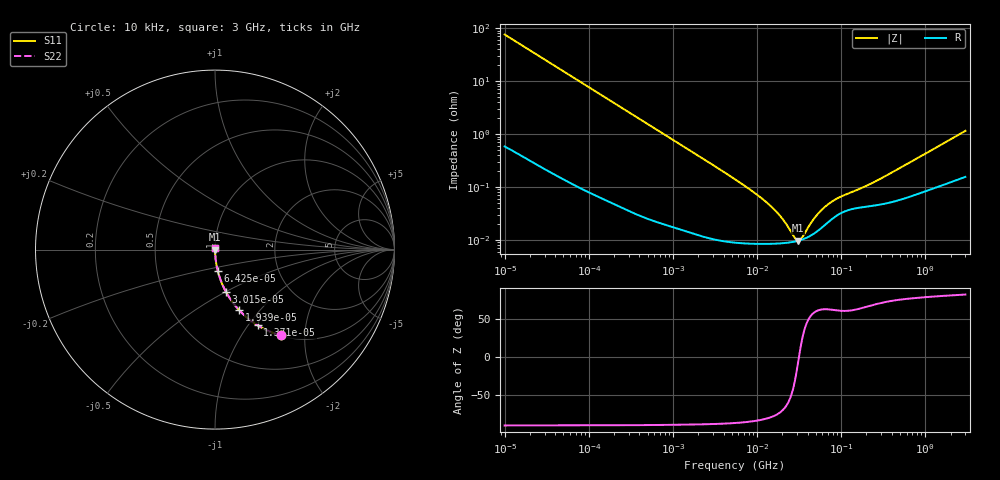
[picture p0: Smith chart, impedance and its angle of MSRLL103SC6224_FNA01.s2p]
! MSRLL103SC6224_FNA01  S-PARAMETER MODEL  ( Standard Model )
! Model Generated by TAIYO YUDEN Corporation (http://www.ty-top.com)
! Version 2.0
! TAIYO YUDEN Control No. 240510
! Copyright(c) 2010 TAIYO YUDEN CO.,LTD. All Rights Reserved.
! Product Description (link to TY-COMPAS)
! https://ds.yuden.co.jp/TYCOMPAS/or/detail?pn=MSRLL103SC6224MFNA01&u=M
! Products Name : Multilayer Ceramic Capacitors
! Characteristics :
!  Capacitance : 0.22 [uF] , Rated Voltage : 10 [V] , TCC : X6S
!  Case Size : 0.52 x 1.0 / 0.02 x 0.039 [mm/inch] , Thickness : 0.3 / 0.012 [mm/inch]
!  (Conditions: Temperature = 25 [degC] , DC Bias Voltage = 0 [V])
! External Node Assignments :
!  1  o---| |---o  2
! GND o---------o GND
! Frequency Range : 10kHz  -  3GHz  [ 401 STEP ]
# MHZ S RI R 50
! Freq[MHz].  S11 Real  S11 Imag  S21 Real  S21 Imag  S12 Real  S12 Imag  S22 Real  S22 Imag
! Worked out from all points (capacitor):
!   401 points, 10 kHz to 3 GHz, reference 50 ohm
!   read as one part in series: C = 210 nF near 10.65 kHz
!   lowest |Z| = 9.75 mohm at 31.02 MHz (marker M1)
!   series resonance near 31.52 MHz, so ESL is about 120 pH
!   S11 on the Smith chart (normalised r, x): 10 kHz: 1.01, -1.52; 13.71 kHz: 1.01, -1.11; 19.39 kHz: 1.01, -0.79; 30.15 kHz: 1.00, -0.51; 64.25 kHz: 1.00, -0.24; 3 GHz: 1.00, +0.02
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0.01  0.3661 -0.4779  0.6339 0.4779  0.6339 0.4779  0.3661 -0.4779
0.013707  0.2368 -0.4211  0.7632 0.4211  0.7632 0.4211  0.2368 -0.4211
0.019389  0.1356 -0.3382  0.8644 0.3382  0.8644 0.3382  0.1356 -0.3382
0.030147  0.062 -0.2368  0.938 0.2368  0.938 0.2368  0.062 -0.2368
0.06425  0.0151 -0.1173  0.9849 0.1173  0.9849 0.1173  0.0151 -0.1173
0.082683  0.00943 -0.0918  0.9906 0.0918  0.9906 0.0918  0.00943 -0.0918
0.199902  0.00196 -0.0385  0.998 0.0385  0.998 0.0385  0.00196 -0.0385
0.683653  0.000341 -0.0114  0.9997 0.0114  0.9997 0.0114  0.000341 -0.0114
5.477226  9.11e-05 -0.0014  0.9999 0.0014  0.9999 0.0014  9.11e-05 -0.0014
9.97066  8.52e-05 -0.000715  0.9999 0.000715  0.9999 0.000715  8.52e-05 -0.000715
15.02209  8.51e-05 -0.000409  0.9999 0.000409  0.9999 0.000409  8.51e-05 -0.000409
20.5901  8.74e-05 -0.000222  0.9999 0.000222  0.9999 0.000222  8.74e-05 -0.000222
28.22191  9.38e-05 -5.63e-05  0.9999 5.63e-05  0.9999 5.63e-05  9.38e-05 -5.63e-05
31.02164  9.72e-05 -8.02e-06  0.9999 8.02e-06  0.9999 8.02e-06  9.72e-05 -8.02e-06
33.04079  0.0001 2.42e-05  0.9999 -2.42e-05  0.9999 -2.42e-05  0.0001 2.42e-05
35.19136  0.000104 5.66e-05  0.9999 -5.66e-05  0.9999 -5.66e-05  0.000104 5.66e-05
45.28751  0.000126 0.000189  0.9999 -0.000189  0.9999 -0.000189  0.000126 0.000189
60.14696  0.000176 0.000342  0.9998 -0.000342  0.9998 -0.000342  0.000176 0.000342
82.4407  0.000267 0.000498  0.9997 -0.000498  0.9997 -0.000498  0.000267 0.000498
205.6994  0.00043 0.000988  0.9996 -0.000988  0.9996 -0.000988  0.00043 0.000988
374.4521  0.000509 0.0017  0.9995 -0.0017  0.9995 -0.0017  0.000509 0.0017
3000  0.00168 0.0114  0.9983 -0.0114  0.9983 -0.0114  0.00168 0.0114
